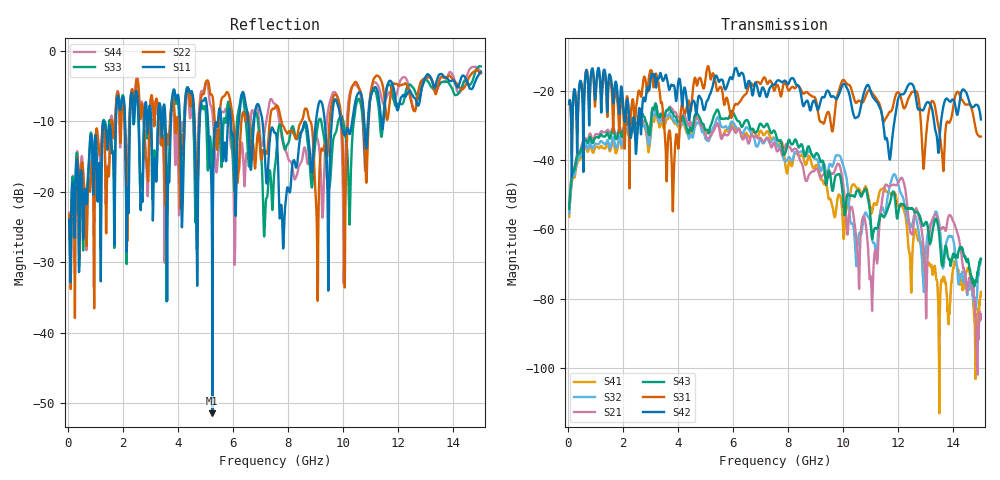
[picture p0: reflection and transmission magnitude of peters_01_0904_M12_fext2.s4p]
# MHZ S RI R 50.00
! FREQ  S11  S12  S13  S14
!  S21  S22  S23  S24
!  S31  S32  S33  S34
!  S41  S42  S43  S44
!  REAL  IMAG  REAL  IMAG  REAL  IMAG  REAL  IMAG
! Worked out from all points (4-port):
!   1496 points, 50 MHz to 15 GHz, reference 50 ohm
!   strongest paths, dB at 50 MHz, 3.79 GHz, 7.53 GHz, 11.27 GHz, 15 GHz:
!     S42: -23.7, -18.4, -18.0, -23.8, -28.3
!     S31: -23.8, -45.4, -19.4, -23.1, -33.2
!     S43: -54.1, -26.2, -31.9, -59.1, -68.5
!     S21: -53.5, -25.2, -35.7, -65.4, -84.4
!     S32: -55.5, -27.6, -34.1, -60.1, -68.8
!     S41: -56.3, -28.1, -34.1, -51.0, -78.0
!   lowest |S11| = -51.4 dB at 5.25 GHz (marker M1), VSWR 1.01, Z = 50.3 - j0.0491 ohm
!   |S11| at or under -10 dB: start of sweep to 1.295 GHz; 1.309 GHz to 1.75 GHz (440.9 MHz wide, 28.8 % of centre); 7.07 GHz to 9.01 GHz (1.94 GHz wide, 24.1 % of centre)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
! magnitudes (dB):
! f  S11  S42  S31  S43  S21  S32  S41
! 50 MHz  -24.0  -23.7  -23.8  -54.1  -53.5  -55.5  -56.3
! 3.02 GHz  -9.1  -16.2  -14.1  -29.6  -28.6  -31.2  -32.3
! 3.82 GHz  -5.9  -18.5  -54.8  -26.6  -25.6  -28.0  -28.6
! 5.25 GHz  -51.4  -19.1  -15.1  -28.7  -32.2  -31.1  -31.7
! 11.02 GHz  -6.2  -20.8  -20.2  -60.2  -75.9  -60.1  -55.3
! 12.13 GHz  -6.5  -21.0  -23.1  -52.6  -45.1  -50.1  -53.3
! 15 GHz  -3.0  -28.3  -33.2  -68.5  -84.4  -68.8  -78.0
